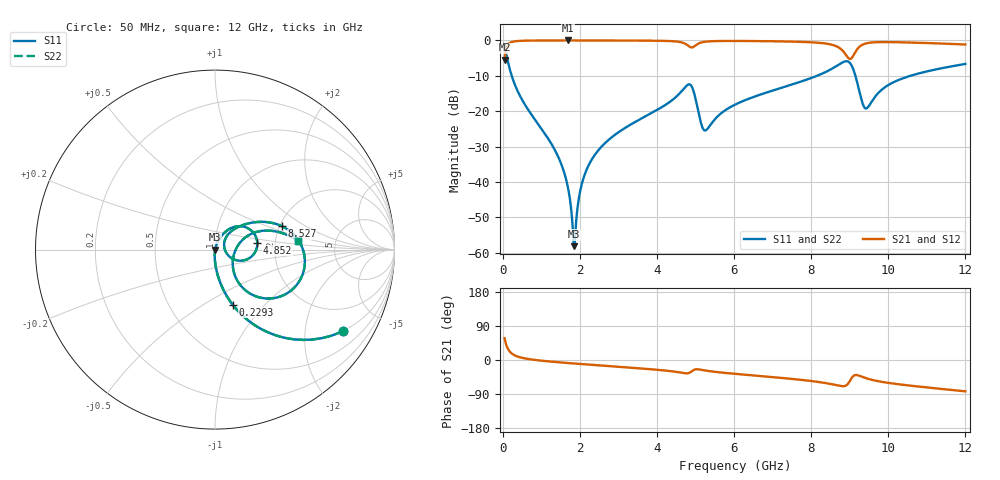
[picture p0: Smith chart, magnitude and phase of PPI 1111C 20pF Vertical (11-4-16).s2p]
# GHz S MA R 50
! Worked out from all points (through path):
!   1601 points, 50 MHz to 12 GHz, reference 50 ohm
!   highest |S21| = -0.01 dB at 1.693 GHz (marker M1); lowest = -5.5 dB at 50 MHz (marker M2)
!   group delay of S21, straight-line fit = 19.8 ps
!   lowest |S11| = -58.2 dB at 1.857 GHz (marker M3), VSWR 1.00, Z = 50.1 - j0.00989 ohm
!   |S11| at or under -10 dB: 234.1 MHz to 8.152 GHz (7.918 GHz wide, 189 % of centre); 9.147 GHz to 10.58 GHz (1.429 GHz wide, 14.5 % of centre)
!   |S22| runs from -58.2 to -1.5 dB; largest |S21 - S12| = 0
!   S11 on the Smith chart (normalised r, x): 50 MHz: 0.99, -3.15; 229.2 MHz: 0.99, -0.68; 4.852 GHz: 1.61, +0.13; 8.527 GHz: 2.05, +0.64; 12 GHz: 2.69, +0.34
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0.05  0.8455 -32.5  0.5338 57.5  0.5338 57.5  0.8455 -32.5
0.1470937  0.472 -62.5  0.8812 27.4  0.8812 27.4  0.472 -62.5
0.22925  0.3224 -72.3  0.9461 17.7  0.9461 17.7  0.3224 -72.3
0.58775  0.121 -85.7  0.9919 4.0  0.9919 4.0  0.121 -85.7
1.386906  0.02601 -93.1  0.9985 -5.5  0.9985 -5.5  0.02601 -93.1
1.693125  0.008284 -89.9  0.9987 -8.0  0.9987 -8.0  0.008284 -89.9
1.857438  0.001234 -4.6  0.9987 -9.3  0.9987 -9.3  0.001234 -4.6
2.044156  0.008981 70.9  0.9985 -10.7  0.9985 -10.7  0.008981 70.9
2.26075  0.01857 73.4  0.9983 -12.4  0.9983 -12.4  0.01857 73.4
2.61925  0.03385 72.4  0.9977 -15.0  0.9977 -15.0  0.03385 72.4
4.038312  0.1066 61.1  0.9889 -26.1  0.9889 -26.1  0.1066 61.1
4.852406  0.2388 9.5  0.8109 -33.2  0.8109 -33.2  0.2388 9.5
5.240781  0.0533 9.0  0.9564 -27.5  0.9564 -27.5  0.0533 9.0
6.025  0.1236 49.1  0.9826 -36.5  0.9826 -36.5  0.1236 49.1
8.019156  0.2965 31.5  0.9397 -55.7  0.9397 -55.7  0.2965 31.5
8.527031  0.3945 19.3  0.8719 -63.7  0.8719 -63.7  0.3945 19.3
8.855656  0.5006 -4.4  0.6761 -69.0  0.6761 -69.0  0.5006 -4.4
9.005031  0.4799 -28.6  0.5466 -55.1  0.5466 -55.1  0.4799 -28.6
9.206687  0.2393 -54.5  0.7659 -40.2  0.7659 -40.2  0.2393 -54.5
9.415812  0.109 -16.4  0.9047 -47.7  0.9047 -47.7  0.109 -16.4
10.01331  0.2361 23.4  0.9468 -60.6  0.9468 -60.6  0.2361 23.4
12  0.4651 6.1  0.8749 -82.7  0.8749 -82.7  0.4651 6.1
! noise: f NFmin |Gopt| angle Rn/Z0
0.05  0.0003681  0.8663  1.2  0.0005915
1.372  0.003732  0.6725  6.996  0.002187
2.701  0.00648  0.6391  13.25  0.003346
4.031  0.01388  0.7373  19.67  0.01027
5.36  0.03717  0.8627  26.26  0.05507
6.682  0.02108  0.7267  31.91  0.01421
8.012  0.03287  0.7883  37.88  0.02864
9.341  0.1045  0.9191  44.15  0.2451
10.67  0.03615  0.7629  48.94  0.02573
12  0.03251  0.7219  53.35  0.01863
